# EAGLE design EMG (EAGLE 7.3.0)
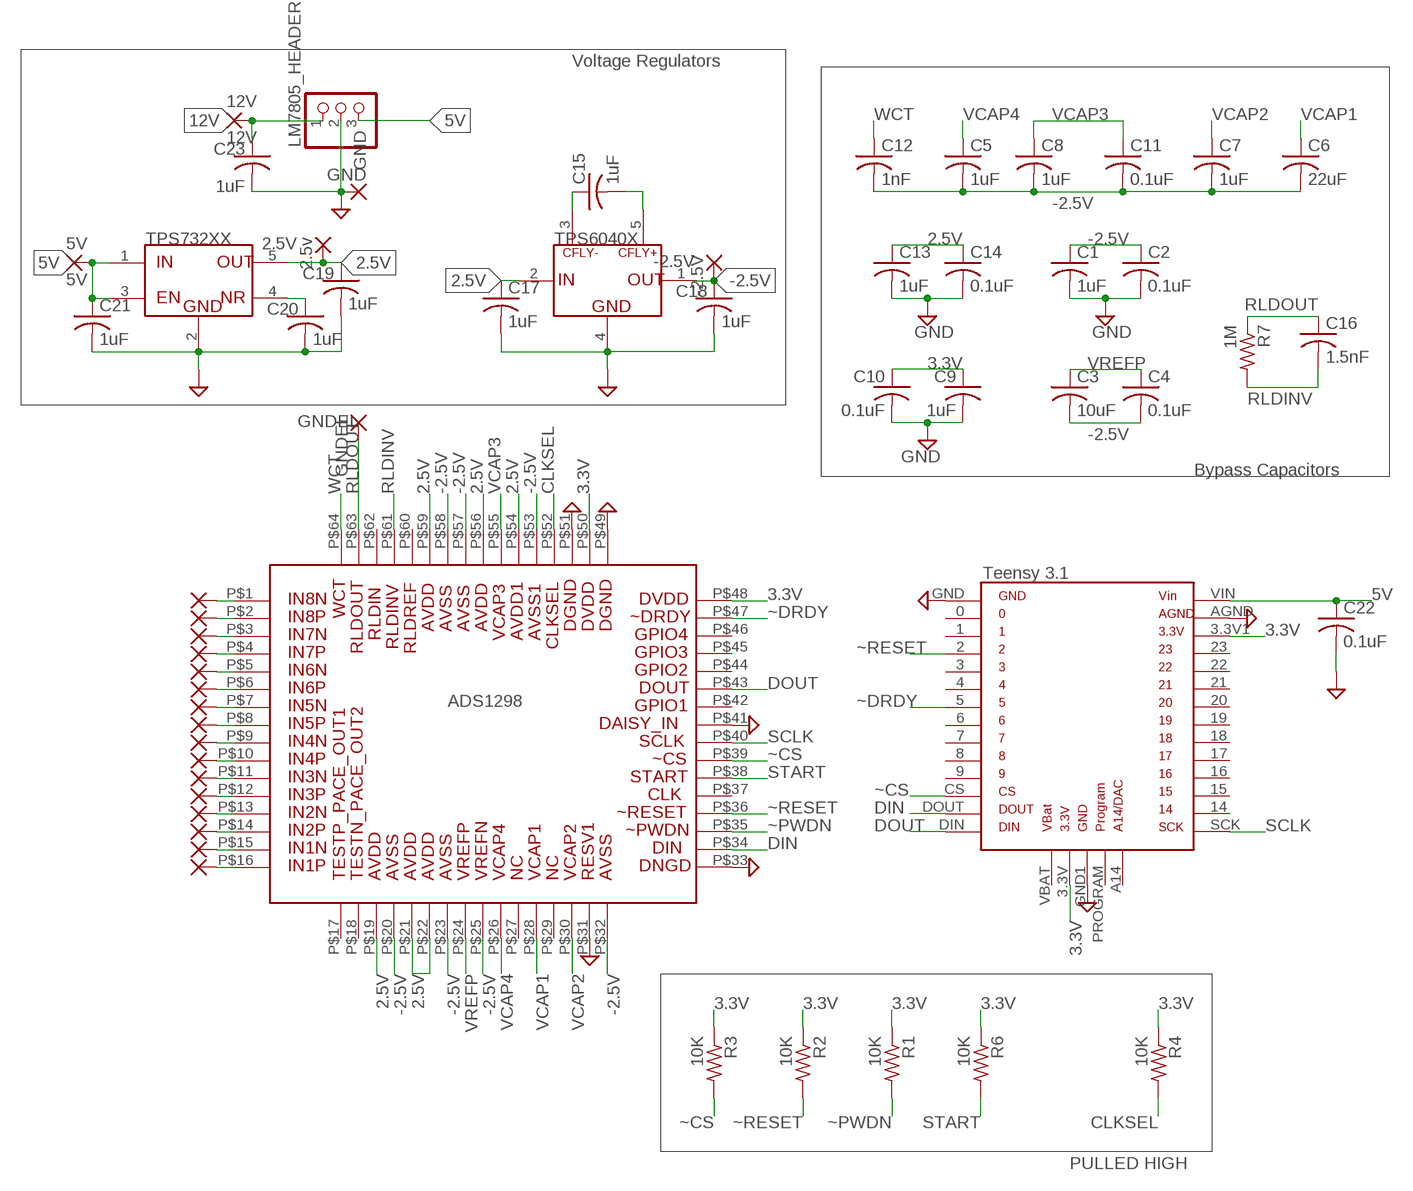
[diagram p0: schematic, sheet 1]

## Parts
2.5V  2.5v  2,54/0,9  [2,54/0,9]
5V  5V  2,54/0,9  [2,54/0,9]
12V  12V  2,54/0,9  [2,54/0,9]
-2.5V  -2.5V  2,54/0,9  [2,54/0,9]
C1  1uF  C-USC0603  [C0603]
C2  0.1uF  C-USC0603  [C0603]
C3  10uF  C-USC0603  [C0603]
C4  0.1uF  C-USC0603  [C0603]
C5  1uF  C-USC0603  [C0603]
C6  22uF  C-USC0603  [C0603]
C7  1uF  C-USC0603  [C0603]
C8  1uF  C-USC0603  [C0603]
C9  1uF  C-USC0603  [C0603]
C10  0.1uF  C-USC0603  [C0603]
C11  0.1uF  C-USC0603  [C0603]
C12  1nF  C-USC0603  [C0603]
C13  1uF  C-USC0603  [C0603]
C14  0.1uF  C-USC0603  [C0603]
C15  1uF  C-USC0603  [C0603]
C16  1.5nF  C-USC0603  [C0603]
C17  1uF  C-USC0603  [C0603]
C18  1uF  C-USC0603  [C0603]
C19  1uF  C-USC0603  [C0603]
C20  1uF  C-USC0603  [C0603]
C21  1uF  C-USC0603  [C0603]
C22  0.1uF  C-USC0603  [C0603]
C23  1uF  C-USC0603  [C0603]
GND  GND  2,54/0,9  [2,54/0,9]
GNDEL  GNDEL  2,54/0,9  [2,54/0,9]
LM7805_HEADER  PINHD-1X3  [1X03]
R1  10K  R-US_R0603  [R0603]
R2  10K  R-US_R0603  [R0603]
R3  10K  R-US_R0603  [R0603]
R4  10K  R-US_R0603  [R0603]
R6  10K  R-US_R0603  [R0603]
R7  1M  R-US_R0603  [R0603]
U$1  ADS1298  [TQFP-64]
U$2  TEENSY3.1  [TEENSY3.1]
U$3  TPS6040X  [SOT23-5]
U$4  TPS732XX  [SOT23-5]
U$5  2X1,6/0,9  [2X1,6/0,9]
U$6  2X1,6/0,9  [2X1,6/0,9]
U$7  2X1,6/0,9  [2X1,6/0,9]
U$8  2X1,6/0,9  [2X1,6/0,9]
U$9  2X1,6/0,9  [2X1,6/0,9]
U$10  2X1,6/0,9  [2X1,6/0,9]
U$11  2X1,6/0,9  [2X1,6/0,9]
U$12  2X1,6/0,9  [2X1,6/0,9]

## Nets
2.5V: 2.5V.1(P) C13.1 C14.1 C17.1 C19.1 U$1.P$19 U$1.P$21 U$1.P$22 U$1.P$54 U$1.P$56 U$1.P$59 U$3.2(IN) U$4.5(OUT)
3.3V: C9.1 C10.1 R1.1 R2.1 R3.1 R4.1 R6.1 U$1.P$48 U$1.P$50 U$2.3.3V U$2.3.3V1
5V: 5V.1(P) C21.1 C22.1 LM7805_HEADER.3 U$2.VIN U$4.1(IN) U$4.3(EN)
12V: 12V.1(P) C23.1 LM7805_HEADER.1
-2.5V: -2.5V.1(P) C1.1 C2.1 C3.2 C4.2 C5.2 C6.2 C7.2 C8.2 C11.2 C12.2 C18.1 U$1.P$20 U$1.P$23 U$1.P$25 U$1.P$32 U$1.P$53 U$1.P$57 U$1.P$58 U$3.1(OUT)
CLKSEL: R4.2 U$1.P$52
DIN: U$1.P$34 U$2.DOUT
DOUT: U$1.P$43 U$2.DIN
GND: C1.2 C2.2 C9.2 C10.2 C13.2 C14.2 C17.2 C18.2 C19.2 C20.2 C21.2 C22.2 C23.2 GND.1(P) LM7805_HEADER.2 U$1.P$31 U$1.P$33 U$1.P$41 U$1.P$49 U$1.P$51 U$2.AGND U$2.GND U$2.GND1 U$3.4(GND) U$4.2(GND)
N$1: U$1.P$1 U$5.1(P)
N$2: U$1.P$2 U$5.2(P1)
N$3: U$1.P$3 U$6.1(P)
N$4: U$1.P$4 U$6.2(P1)
N$5: U$1.P$5 U$7.1(P)
N$6: U$1.P$6 U$7.2(P1)
N$7: U$1.P$7 U$8.1(P)
N$8: U$1.P$8 U$8.2(P1)
N$9: U$1.P$9 U$9.1(P)
N$10: U$1.P$10 U$9.2(P1)
N$11: U$1.P$11 U$10.1(P)
N$12: U$1.P$12 U$10.2(P1)
N$13: U$1.P$13 U$11.1(P)
N$14: U$1.P$14 U$11.2(P1)
N$15: U$1.P$15 U$12.1(P)
N$16: U$1.P$16 U$12.2(P1)
N$17: C15.1 U$3.3(CFLY-)
N$18: C15.2 U$3.5(CFLY+)
N$20: C20.1 U$4.4(NR)
RLDINV: C16.2 R7.2 U$1.P$61
RLDOUT: C16.1 GNDEL.1(P) R7.1 U$1.P$63
SCLK: U$1.P$40 U$2.SCK
START: R6.2 U$1.P$38
VCAP1: C6.1 U$1.P$28
VCAP2: C7.1 U$1.P$30
VCAP3: C8.1 C11.1 U$1.P$55
VCAP4: C5.1 U$1.P$26
VREFP: C3.1 C4.1 U$1.P$24
WCT: C12.1 U$1.P$64
~CS: R3.2 U$1.P$39 U$2.CS
~DRDY: U$1.P$47 U$2.5
~PWDN: R1.2 U$1.P$35
~RESET: R2.2 U$1.P$36 U$2.2
Unconnected: U$1.P$17 U$1.P$18 U$1.P$27 U$1.P$29 U$1.P$37 U$1.P$42 U$1.P$44 U$1.P$45 U$1.P$46 U$1.P$60 U$1.P$62 U$2.0 U$2.1 U$2.3 U$2.4 U$2.6 U$2.7 U$2.8 U$2.9 U$2.14 U$2.15 U$2.16 U$2.17 U$2.18 U$2.19 U$2.20 U$2.21 U$2.22 U$2.23 U$2.A14 U$2.PROGRAM U$2.VBAT

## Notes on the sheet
- Voltage Regulators
- Bypass Capacitors
- PULLED HIGH

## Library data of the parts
2.5V 5V 12V -2.5V GND GNDEL = wirepad:2,54/0,9: THROUGH-HOLE PAD
C1-C23 = adafruit:C-US: CAPACITOR, American symbol
LM7805_HEADER = pinhead:PINHD-1X3: PIN HEADER
R1-R4 R6 R7 = adafruit:R-US_: RESISTOR, American symbol
U$1 = ADS1298:ADS1298: ADS1298 Chris Yim - May 2015
U$2 = Teensy3.1:TEENSY3.1: Teensy 3.1 Chris Yim - May 2015
U$3 = sot23-5:TPS6040X
U$4 = sot23-5:TPS732XX
U$5-U$12 = wirepad:2X1,6/0,9

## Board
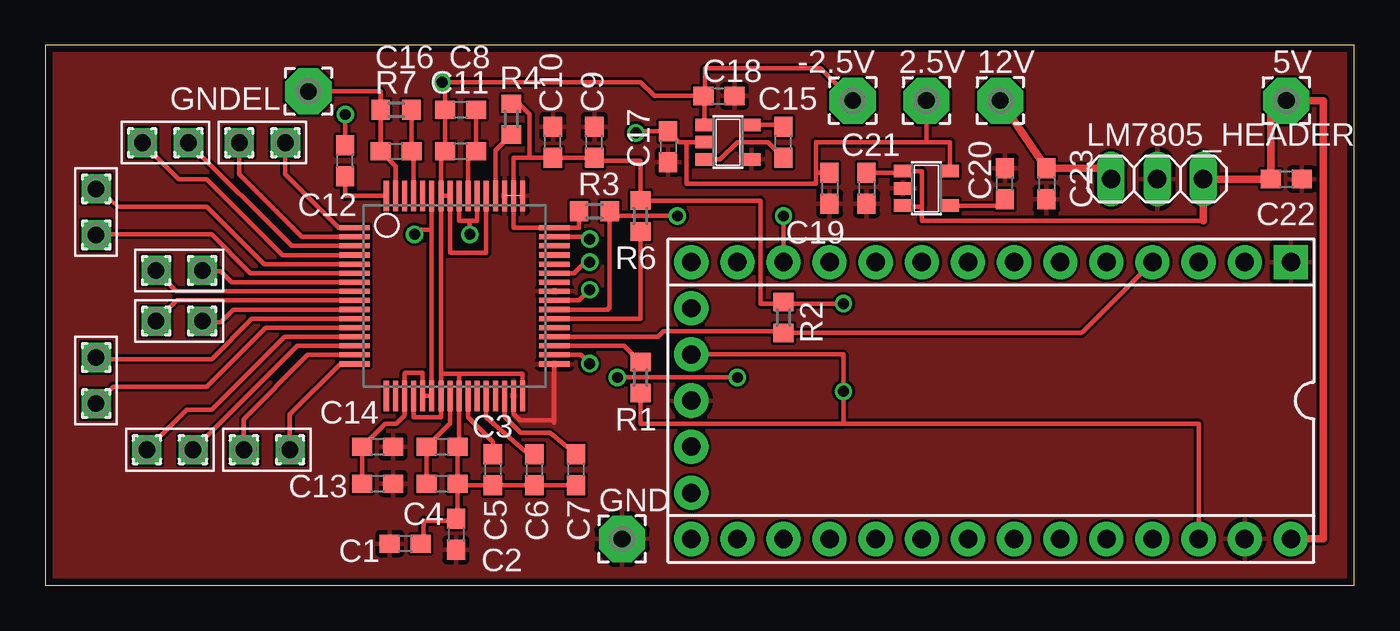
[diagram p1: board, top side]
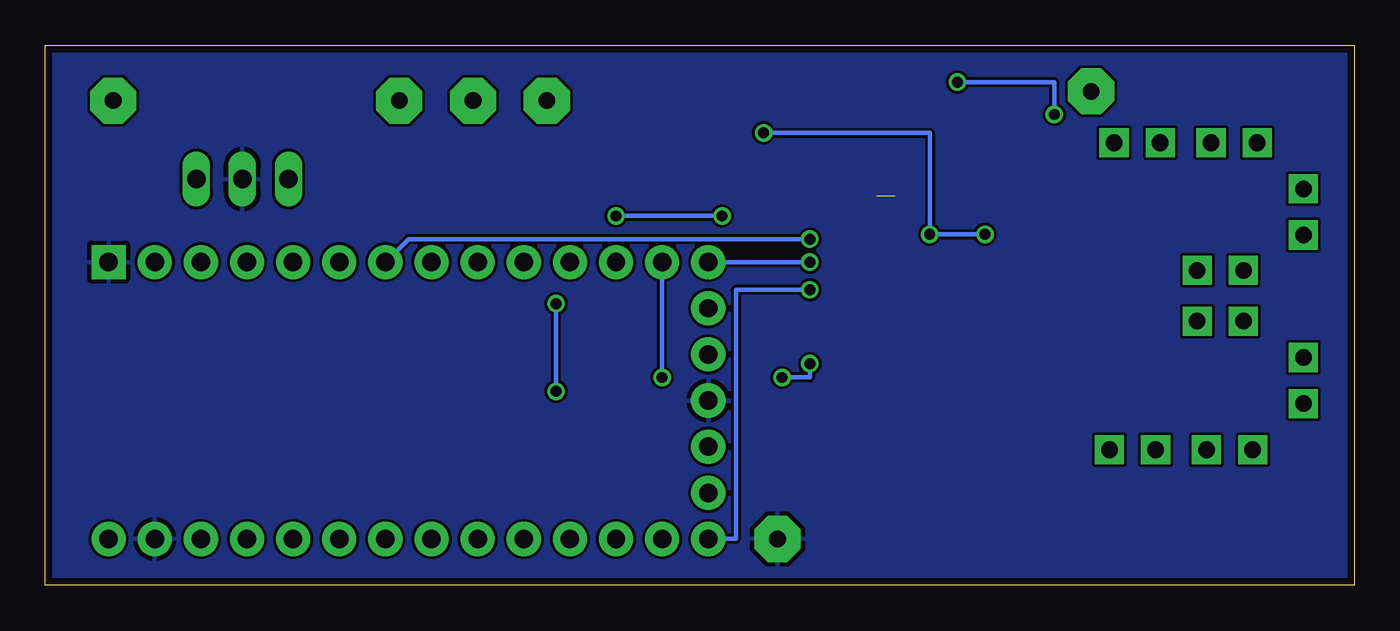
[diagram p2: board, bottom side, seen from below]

Size 72.06 x 29.71 mm. Coordinates in mm from the lower left corner, seen from the top.
Outline: 0,0 72.06,0 72.06,29.71 0,29.71 0,0
Copper layers (1*16): Top 0.0356mm / dielectric 1.5011mm / Bottom 0.0356mm
Design rules "LaenPCBOrder": minimum track width 6mil, minimum drill 13mil, track to track 6mil, track to pad 6mil, pad to pad 6mil, via to via 6mil, smd to smd 6mil, copper to edge 15mil, drill to drill 6mil, minimum pad ring 7mil, minimum via ring 7mil, stop-mask expansion 3mil, vias tented up to drill 0mil, thermal gap 10mil

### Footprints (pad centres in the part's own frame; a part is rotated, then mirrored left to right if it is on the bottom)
2,54/0,9 = drill 0.914 pad 2.54 octagon: 1 0,0
C0603 = smd 1.1 x 1: 1 -0.85,0; 2 0.85,0
1X03 = drill 1.016 long: 1 -2.54,0; 2 0,0; 3 2.54,0
R0603 = smd 1 x 1.1: 1 -0.85,0; 2 0.85,0
TQFP-64 = smd 1.676 x 0.279: P$1 -5.58,3.67; P$2 -5.58,3.17; P$3 -5.58,2.67; P$4 -5.58,2.17; P$5 -5.58,1.67; P$6 -5.58,1.17; P$7 -5.58,0.67; P$8 -5.58,0.17; P$9 -5.58,-0.33; P$10 -5.58,-0.83; P$11 -5.58,-1.33; P$12 -5.58,-1.83; P$13 -5.58,-2.33; P$14 -5.58,-2.83; P$15 -5.58,-3.33; P$16 -5.58,-3.83; P$33 5.42,-3.83; P$34 5.42,-3.33; P$35 5.42,-2.83; P$36 5.42,-2.33; P$37 5.42,-1.83; P$38 5.42,-1.33; P$39 5.42,-0.83; P$40 5.42,-0.33; P$41 5.42,0.17; P$42 5.42,0.67; P$43 5.42,1.17; P$44 5.42,1.67; P$45 5.42,2.17; P$46 5.42,2.67; P$47 5.42,3.17; P$48 5.42,3.67 | smd 0.279 x 1.676: P$17 -3.83,-5.58; P$18 -3.33,-5.58; P$19 -2.83,-5.58; P$20 -2.33,-5.58; P$21 -1.83,-5.58; P$22 -1.33,-5.58; P$23 -0.83,-5.58; P$24 -0.33,-5.58; P$25 0.17,-5.58; P$26 0.67,-5.58; P$27 1.17,-5.58; P$28 1.67,-5.58; P$29 2.17,-5.58; P$30 2.67,-5.58; P$31 3.17,-5.58; P$32 3.67,-5.58; P$49 3.67,5.42; P$50 3.17,5.42; P$51 2.67,5.42; P$52 2.17,5.42; P$53 1.67,5.42; P$54 1.17,5.42; P$55 0.67,5.42; P$56 0.17,5.42; P$57 -0.33,5.42; P$58 -0.83,5.42; P$59 -1.33,5.42; P$60 -1.83,5.42; P$61 -2.33,5.42; P$62 -2.83,5.42; P$63 -3.33,5.42; P$64 -3.83,5.42
TEENSY3.1 = drill 1.016 pad 1.88: 0 -13.97,-7.62; 1 -11.43,-7.62; 2 -8.89,-7.62; 3 -6.35,-7.62; 3.3V 16.51,-2.54; 3.3V1 -11.43,7.62; 4 -3.81,-7.62; 5 -1.27,-7.62; 6 1.27,-7.62; 7 3.81,-7.62; 8 6.35,-7.62; 9 8.89,-7.62; 14 13.97,7.62; 15 11.43,7.62; 16 8.89,7.62; 17 6.35,7.62; 18 3.81,7.62; 19 1.27,7.62; 20 -1.27,7.62; 21 -3.81,7.62; 22 -6.35,7.62; 23 -8.89,7.62; A14 16.51,5.08; AGND -13.97,7.62; CS 11.43,-7.62; DIN 16.51,-7.62; DOUT 13.97,-7.62; GND1 16.51,0; PROGRAM 16.51,2.54; SCK 16.51,7.62; VBAT 16.51,-5.08; VIN -16.51,7.62 | drill 1.016 pad 1.88 square: GND -16.51,-7.62
SOT23-5 = smd 0.69 x 0.99: 1 -0.95,-1.29; 2 0,-1.29; 3 0.95,-1.29; 4 0.95,1.3; 5 -0.95,1.3
2X1,6/0,9 = drill 0.914 pad 1.6 square: 1 0,0; 2 0,-2.54

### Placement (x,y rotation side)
2.5V  48.51,26.67 0 top
5V  68.33,26.67 0 top
12V  52.58,26.67 0 top
-2.5V  44.45,26.67 0 top
C1  19.81,2.29 180 top
C2  22.61,2.79 270 top
C3  21.84,7.62 0 top
C4  21.84,5.59 0 top
C5  24.64,6.35 270 top
C6  26.92,6.35 270 top
C7  29.21,6.35 270 top
C8  22.86,23.88 180 top
C9  30.23,24.38 90 top
C10  27.94,24.38 90 top
C11  22.86,26.16 180 top
C12  16.51,23.37 90 top
C13  18.29,5.59 0 top
C14  18.29,7.62 0 top
C15  40.64,24.38 90 top
C16  19.3,23.88 0 top
C17  34.29,24.13 270 top
C18  37.08,26.92 0 top
C19  43.18,21.84 270 top
C20  52.83,22.1 90 top
C21  45.21,21.84 270 top
C22  68.33,22.35 0 top
C23  55.12,22.1 270 top
GND  31.75,2.54 0 top
GNDEL  14.48,27.18 0 top
LM7805_HEADER  61.21,22.35 0 top
R1  32.77,11.43 90 top
R2  40.64,14.73 270 top
R3  30.23,20.57 0 top
R4  25.65,25.65 270 top
R6  32.77,20.32 270 top
R7  19.3,26.16 0 top
U$1  22.61,16 0 top
U$2  52.07,10.16 180 top
U$3  37.59,24.38 270 top
U$4  48.51,21.84 270 top
U$5  13.22,24.35 270 top
U$6  7.87,24.35 270 top
U$7  2.79,21.81 0 top
U$8  8.64,17.32 270 top
U$9  6.1,14.53 90 top
U$10  2.79,12.53 0 top
U$11  5.59,7.45 90 top
U$12  10.93,7.45 90 top

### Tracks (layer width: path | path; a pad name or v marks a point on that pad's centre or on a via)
2.5V  (via drill 0.6)
  Top 0.254: C13.1 C14.1 18.71,8.89 19.3,8.89 19.78,9.36 U$1.P$19 19.78,11.65 19.81,11.68 20.78,11.68 U$1.P$21 U$1.P$22 21.28,19.56 | 21.28,19.56 U$1.P$59 | U$1.P$56 22.78,20.07 23.37,20.07 | U$1.P$54 23.78,20.07 23.37,20.07 | 23.37,20.07 v23.37,19.3 | 21.28,19.56 20.57,19.56 v20.32,19.3 | 42.42,22.69 42.42,22.1 35.31,22.1 35.31,24.38 U$3.2 34.89,24.38 C17.1 32.51,24.98 v32.51,24.89 | 42.42,22.69 42.42,24.38 48.51,24.38 | 48.51,24.38 49.81,24.38 U$4.5 | C19.1 42.42,22.69 | 2.5V.1 48.51,24.38
  Bottom 0.254: v20.32,19.3 v23.37,19.3 23.37,24.89 v32.51,24.89
3.3V  (via drill 0.6)
  Top 0.254: U$2.3.3V1 63.5,8.89 43.94,8.89 | 43.94,8.89 v43.94,10.67 43.94,12.7 U$2.3.3V | v43.94,15.49 40.64,15.49 | R3.1 29.38,19.67 U$1.P$48 25.78,19.67 U$1.P$50 25.78,23.53 26.67,23.53 | 26.67,23.53 C10.1 C9.1 30.23,23.37 32.77,23.37 R6.1 | R1.1 32.77,8.89 43.94,8.89 | R6.1 39.37,21.17 39.37,15.49 40.64,15.49 | 40.64,15.49 R2.1 | R4.1 26.07,26.5 26.67,25.91 26.67,23.53 | R6.1 32.77,21.08
  Bottom 0.254: v43.94,10.67 v43.94,15.49
5V
  Top 0.254: C21.1 47.22,22.69 U$4.1 48.26,22.79 48.26,20.83 | 48.26,20.83 47.22,20.83 U$4.3 | 63.75,20.07 48.26,20.07 48.26,20.83
  Top 0.406: U$2.VIN 70.36,2.54 70.36,26.67 5V.1 67.48,26.67 C22.1 LM7805_HEADER.3 63.75,20.07
12V
  Top 0.406: 12V.1 C23.1 58.67,22.95 LM7805_HEADER.1
-2.5V  (via drill 0.6)
  Top 0.254: U$1.P$20 20.29,9.23 21.78,9.23 U$1.P$23 21.78,11.63 | 21.78,11.63 U$1.P$58 | 22.79,11.63 U$1.P$25 22.78,7.62 C3.2 C4.2 | 22.79,11.63 21.78,11.63 | U$1.P$32 26.29,11.63 22.79,11.63 | C4.2 22.69,3.73 C2.1 22.61,3.56 20.83,3.56 20.83,2.29 C1.1 | C4.2 22.78,5.5 C5.2 C6.2 C7.2 | U$1.P$53 24.28,18.29 22.28,18.29 U$1.P$57 U$1.P$58 | U$1.P$58 21.78,23.64 C8.2 C11.2 22.01,27.69 v21.84,27.69 32.77,27.69 33.53,26.92 36.32,26.92 | C18.1 36.3,26.86 U$3.1 36.3,26.9 36.32,26.92 | v16.51,25.91 C12.2 | 36.32,26.92 36.32,28.45 42.67,28.45 -2.5V.1
  Bottom 0.254: v16.51,25.91 16.51,27.69 v21.84,27.69
CLKSEL
  Top 0.254: U$1.P$52 24.78,23.93 R4.2
DIN  (via drill 0.6)
  Top 0.254: U$1.P$34 29.49,12.67 v29.97,12.19 | v31.5,11.43 v38.1,11.43
  Bottom 0.254: v29.97,12.19 29.97,11.43 v31.5,11.43 | v38.1,11.43 U$2.DOUT
DOUT  (via drill 0.6)
  Top 0.254: U$1.P$43 29.11,17.17 29.72,17.78 v29.97,17.78
  Bottom 0.254: v29.97,17.78 U$2.DIN
GND  (1 unrouted)
  Top 0.254: U$1.P$31 25.78,9.42 26.14,9.07 27.89,9.07 28.02,8.94 28.02,12.16 U$1.P$33
  pour Bottom: 0,0 72.14,0 72.14,1.52 72.14,27.94 72.14,29.72 0,29.72
  pour Top: 72.14,0 72.14,29.72 0,29.72 0,0
N$1
  Top 0.254: U$1.P$1 16.14,19.67 13.21,22.61 13.21,24.34 U$5.1
N$2
  Top 0.254: U$1.P$2 14.1,19.17 10.67,22.61 10.67,24.34 U$5.2
N$3
  Top 0.254: U$1.P$3 13.55,18.67 U$6.1
N$4
  Top 0.254: U$1.P$4 13.07,18.17 8.89,22.35 7.33,22.35 U$6.2
N$5
  Top 0.254: U$1.P$5 12.05,17.67 8.89,20.83 4.03,20.83 U$7.1
N$6
  Top 0.254: U$1.P$6 11.28,17.17 9.14,19.3 2.32,19.3 U$7.2
N$7
  Top 0.254: U$1.P$7 10.25,16.67 9.65,17.27 8.69,17.27 U$8.1
N$8
  Top 0.254: U$1.P$8 7.2,16.17 U$8.2
N$9
  Top 0.254: U$1.P$9 7.24,15.67 U$9.1
N$10
  Top 0.254: U$1.P$10 10.35,15.17 9.65,14.48 8.69,14.48 U$9.2
N$11
  Top 0.254: U$1.P$11 11.37,14.67 9.14,12.45 2.37,12.45 U$10.1
N$12
  Top 0.254: U$1.P$12 12.14,14.17 8.89,10.92 3.72,10.92 U$10.2
N$13
  Top 0.254: U$1.P$13 13.16,13.67 9.14,9.65 7.79,9.65 U$11.1
N$14
  Top 0.254: U$1.P$14 13.85,13.17 U$11.2
N$15
  Top 0.254: U$1.P$15 14.45,12.67 10.92,9.14 U$12.1
N$16
  Top 0.254: U$1.P$16 16.24,12.17 13.46,9.4 U$12.2
N$17
  Top 0.254: U$3.3 37.15,23.43 38.1,24.38 39.79,24.38 C15.1
N$18
  Top 0.254: U$3.5 40.64,25.33 C15.2
N$20
  Top 0.254: U$4.4 52.58,20.89 C20.1
RLDINV
  Top 0.254: U$1.P$61 20.28,23.75 C16.2 R7.2
RLDOUT
  Top 0.254: U$1.P$63 19.28,23.05 C16.1 R7.1 18.45,27.18 GNDEL.1
SCLK  (via drill 0.6)
  Top 0.254: U$1.P$40 29.39,15.67 v29.97,16.26
  Bottom 0.254: v29.97,16.26 34.04,16.26 34.04,2.54 U$2.SCK
START
  Top 0.254: U$1.P$38 32.77,14.67 R6.2
VCAP1
  Top 0.254: U$1.P$28 24.28,9.25 26.42,7.37 26.76,7.37 C6.1
VCAP2
  Top 0.254: U$1.P$30 25.28,9.27 26.16,8.38 27.77,8.38 C7.1
VCAP3
  Top 0.254: U$1.P$55 23.28,23.44 C8.1 C11.1
VCAP4
  Top 0.254: U$1.P$26 23.28,9.24 24.64,7.87 C5.1
VREFP
  Top 0.254: U$1.P$24 22.28,8.9 C3.1 C4.1
WCT
  Top 0.254: U$1.P$64 16.51,21.42 C12.1
~CS  (via drill 0.6)
  Top 0.254: U$1.P$39 30.99,15.17 30.99,15.24 31.08,15.24 R3.2 31.33,20.32 v34.8,20.32 | v40.64,20.32 U$2.CS
  Bottom 0.254: v40.64,20.32 v34.8,20.32
~DRDY  (via drill 0.6)
  Top 0.254: U$1.P$47 29.85,19.17 v29.97,19.05
  Bottom 0.254: v29.97,19.05 52.07,19.05 U$2.5
~PWDN
  Top 0.254: U$1.P$35 31.87,13.17 R1.2
~RESET
  Top 0.254: U$1.P$36 33.74,13.67 34.04,13.97 40.55,13.97 R2.2 57.06,13.88 U$2.2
